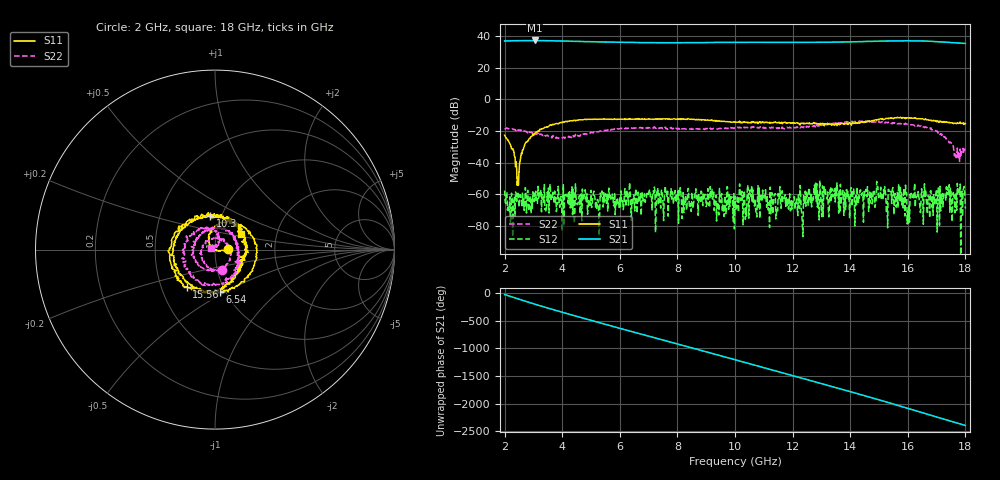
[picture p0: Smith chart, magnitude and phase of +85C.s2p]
!Agilent Technologies,E8361C,US49010292,A.09.42.06
!Agilent E8361C: A.09.42.06
!Date: Wednesday, June 03, 2026 22:47:00
!Correction: S11(Full 2 Port(1,2))
!S21(Full 2 Port(1,2))
!S12(Full 2 Port(1,2))
!S22(Full 2 Port(1,2))
!S2P File: Measurements: S11, S21, S12, S22:
# Hz S  dB  R 50
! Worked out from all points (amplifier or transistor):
!   801 points, 2 GHz to 18 GHz, reference 50 ohm
!   highest |S21| = 37.2 dB at 3.04 GHz (marker M1)
!   |S21| within 3 dB of that: start of sweep to end of sweep
!   unconditionally stable (mu >= 1): start of sweep to end of sweep
!   at 4.66 GHz: K = 6.89, MAG = 36.8 dB, |S12| = -59.8 dB
!   at 10 GHz: K = 8.77, MAG = 36.3 dB, |S12| = -61.3 dB
!   at 18 GHz: K = 23.78, MAG = 35.4 dB, |S12| = -69.1 dB
!   S11 on the Smith chart (normalised r, x): 2 GHz: 1.16, +0.01; 6.54 GHz: 0.94, -0.47; 10.3 GHz: 0.89, +0.34; 15.56 GHz: 0.67, -0.30; 18 GHz: 1.32, +0.24
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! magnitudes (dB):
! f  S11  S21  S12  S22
! 2 GHz  -22.7  36.9  -57.7  -18.3
! 2.22 GHz  -29.7  37.0  -74.1  -18.9
! 2.46 GHz  -50.6  37.1  -61.6  -19.5
! 2.66 GHz  -30.9  37.1  -62.9  -19.7
! 3.04 GHz  -22.2  37.2  -59.4  -21.2
! 4.68 GHz  -12.9  36.6  -76.8  -22.5
! 6.54 GHz  -12.6  35.9  -59.3  -18.1
! 7.34 GHz  -12.5  35.8  -66.9  -18.2
! 9.22 GHz  -13.4  35.9  -63.1  -18.8
! 10 GHz  -14.3  36.0  -61.3  -18.1
! 10.16 GHz  -13.7  36.0  -53.5  -17.5
! 10.3 GHz  -14.5  36.0  -58.1  -18.4
! 11.58 GHz  -15.1  36.0  -64.5  -18.0
! 12.38 GHz  -15.6  36.0  -60.8  -17.9
! 12.68 GHz  -15.5  36.0  -61.8  -17.0
! 15.34 GHz  -12.2  36.9  -56.9  -14.9
! 15.56 GHz  -11.6  36.9  -59.5  -15.2
! 15.98 GHz  -11.6  37.0  -78.8  -15.8
! 16.16 GHz  -11.9  36.9  -61.9  -16.1
! 17.02 GHz  -13.8  36.4  -83.9  -20.5
! 17.72 GHz  -14.8  35.6  -53.1  -30.8
! 18 GHz  -15.4  35.3  -69.1  -32.1
